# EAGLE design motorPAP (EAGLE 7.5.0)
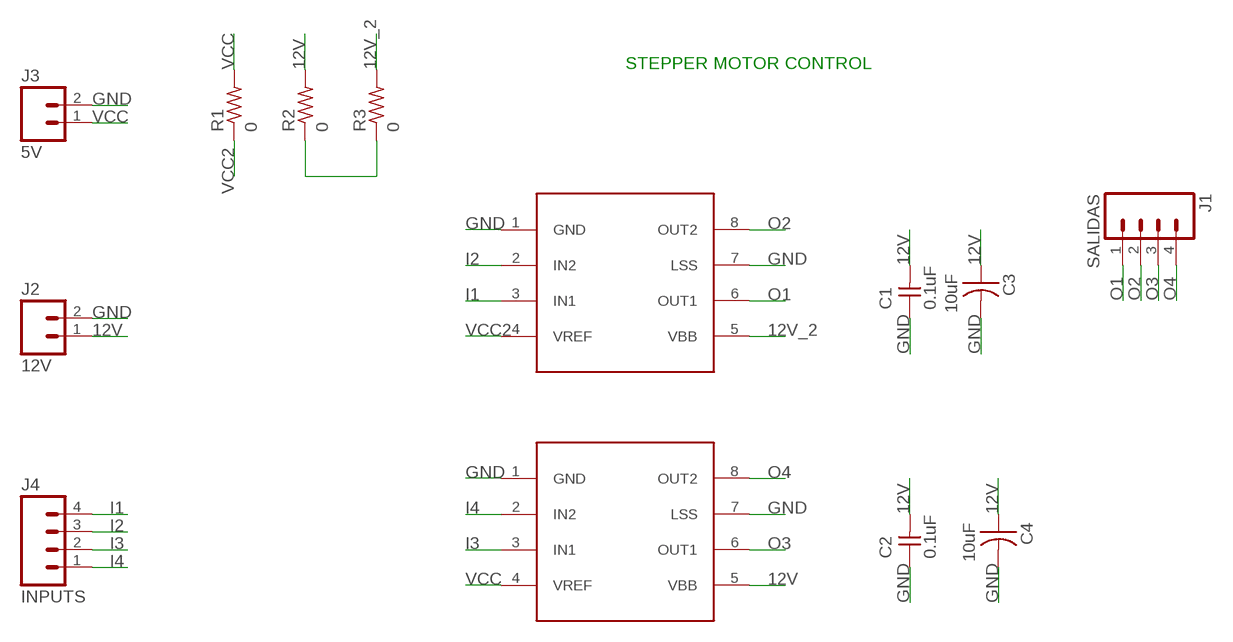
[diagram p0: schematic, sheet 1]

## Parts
C1  0.1uF  CAP-UNPOLARIZEDFAB  [C1206FAB]
C2  0.1uF  CAP-UNPOLARIZEDFAB  [C1206FAB]
C3  10uF  CAP-US1206FAB  [C1206FAB]
C4  10uF  CAP-US1206FAB  [C1206FAB]
J1  SALIDAS  M04PTH  [1X04]
J2  12V  M025MM  [SCREWTERMINAL-5MM-2]
J3  5V  M02PTH  [1X02]
J4  INPUTS  M04PTH  [1X04]
R1  0  RES-US1206FAB  [R1206FAB]
R2  0  RES-US1206FAB  [R1206FAB]
R3  0  RES-US1206FAB  [R1206FAB]
U$1  A4953-H-BRIDGE-MOTOR-DRIVER  [SOIC8]
U$2  A4953-H-BRIDGE-MOTOR-DRIVER  [SOIC8]

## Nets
12V: C1.2 C2.2 C3.1 C4.1 J2.1 R2.2 U$2.5(VBB)
12V_2: R3.2 U$1.5(VBB)
GND: C1.1 C2.1 C3.2 C4.2 J2.2 J3.2 U$1.1(GND) U$1.7(LSS) U$2.1(GND) U$2.7(LSS)
I1: J4.4 U$1.3(IN1)
I2: J4.3 U$1.2(IN2)
I3: J4.2 U$2.3(IN1)
I4: J4.1 U$2.2(IN2)
N$1: R2.1 R3.1
O1: J1.1 U$1.6(OUT1)
O2: J1.2 U$1.8(OUT2)
O3: J1.3 U$2.6(OUT1)
O4: J1.4 U$2.8(OUT2)
VCC: J3.1 R1.2 U$2.4(VREF)
VCC2: R1.1 U$1.4(VREF)

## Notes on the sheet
- STEPPER MOTOR CONTROL

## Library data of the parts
C1 C2 = fab:CAP-UNPOLARIZED
C3 C4 = fab:CAP-US
J1 J4 = SparkFun-Connectors:M04: Header 4 Standard 4-pin 0.1" header. Use with straight break away headers (SKU : PRT-00116), right angle break away headers (PRT-00553), swiss pins (PRT-00743), machine pins (PRT-00117), and female headers (PRT-00115). Molex polarized connector foot print use with SKU : PRT-08231 with associated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; PROD_ID: CONN-09696
J2 = SparkFun-Connectors:M02: Standard 2-pin 0.1" header. Use with; STOREFRONT_ID: PRT-08432
J3 = SparkFun-Connectors:M02: Standard 2-pin 0.1" header. Use with
R1-R3 = fab:RES-US: Resistor (US Symbol)
U$1 U$2 = fab:A4953-H-BRIDGE-MOTOR-DRIVER

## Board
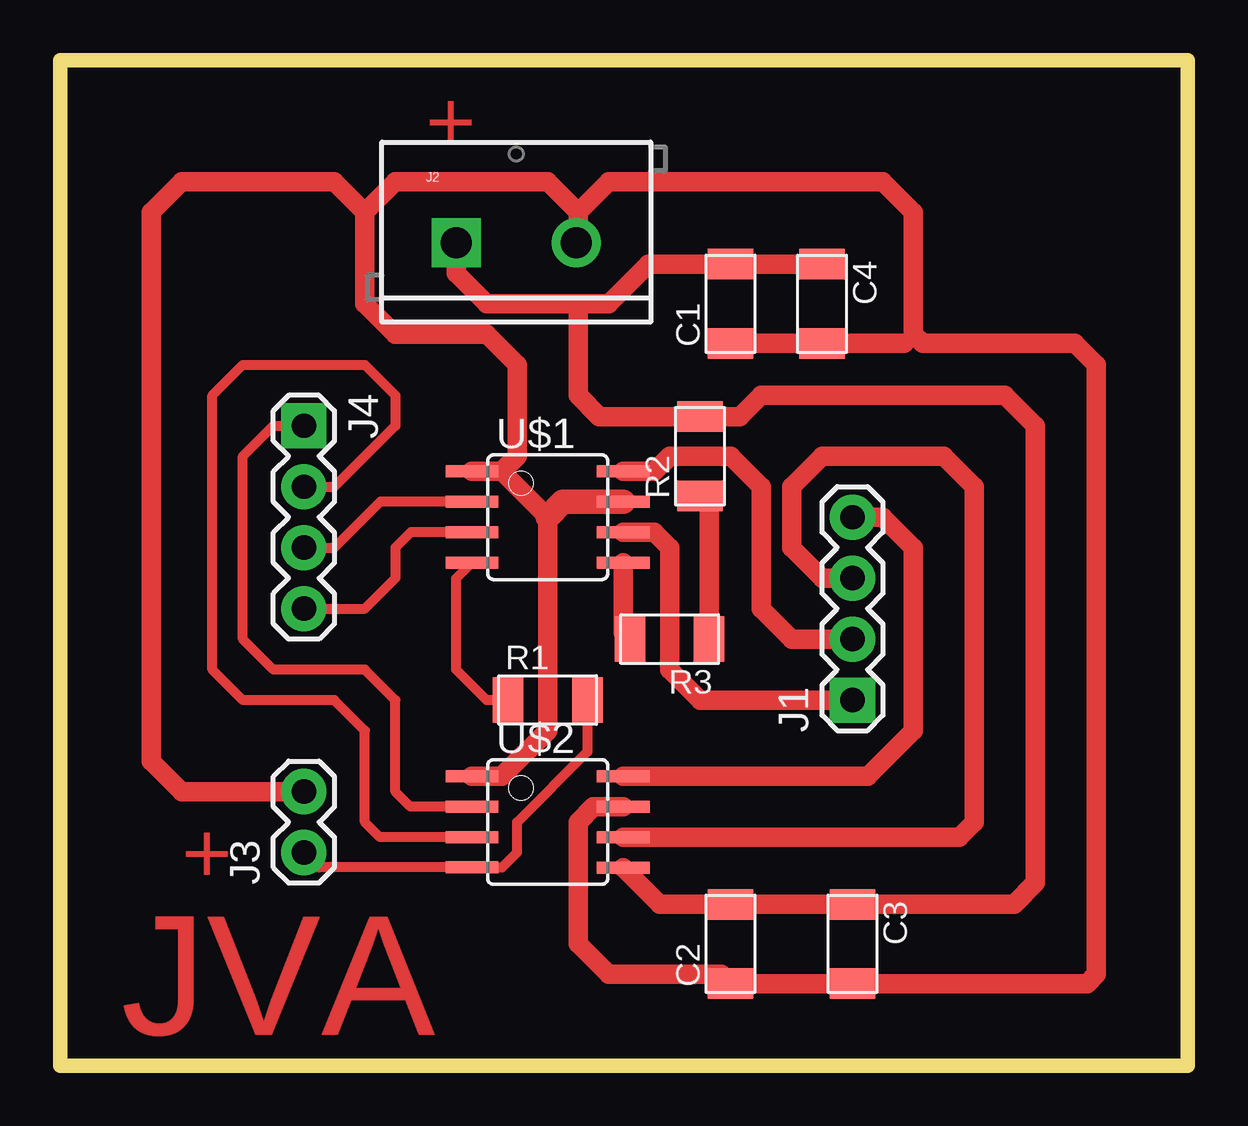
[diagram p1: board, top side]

Size 46.99 x 41.91 mm. Coordinates in mm from the lower left corner, seen from the top.
Outline: 0,41.91 46.99,41.91 46.99,0 0,0 0,41.91
Copper layers (1*16): Top 0.035mm / dielectric 1.5mm / Bottom 0.035mm
Design rules "default": minimum track width 10mil, minimum drill 24mil, track to track 8mil, track to pad 8mil, pad to pad 8mil, via to via 8mil, smd to smd 8mil, copper to edge 40mil, drill to drill 8mil, minimum pad ring 10mil, minimum via ring 8mil, stop-mask expansion 4mil, vias tented up to drill 0mil, thermal gap 10mil

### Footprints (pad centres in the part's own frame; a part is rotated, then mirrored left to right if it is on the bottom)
C1206FAB = smd 1.27 x 1.905: 1 -1.651,0; 2 1.651,0
1X04 = drill 1.016 pad 1.88 square: 1 0,0 | drill 1.016 pad 1.88: 2 2.54,0; 3 5.08,0; 4 7.62,0
SCREWTERMINAL-5MM-2 = drill 1.3 pad 2.032 square: 1 0,0 | drill 1.3 pad 2.032: 2 5,0
1X02 = drill 1.016 pad 1.88: 1 0,0; 2 2.54,0
R1206FAB = smd 1.27 x 1.905: 1 -1.651,0; 2 1.651,0
SOIC8 = smd 0.5 x 2.2: 1 -1.905,-3.154; 2 -0.645,-3.154; 3 0.625,-3.154; 4 1.895,-3.154; 5 1.905,3.154; 6 0.635,3.154; 7 -0.635,3.154; 8 -1.905,3.154

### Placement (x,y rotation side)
C1  27.94,31.75 90 top
C2  27.94,5.08 90 top
C3  33.02,5.08 270 top
C4  31.75,31.75 270 top
J1  33.02,15.24 90 top
J2  16.51,34.29 0 top
J3  10.16,8.89 90 top
J4  10.16,26.67 270 top
R1  20.32,15.24 0 top
R2  26.67,25.4 90 top
R3  25.4,17.78 180 top
U$1  20.32,22.86 270 top
U$2  20.32,10.16 270 top

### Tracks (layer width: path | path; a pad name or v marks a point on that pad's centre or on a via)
12V
  Top 0.813: U$2.5 25,6.73 C2.2 C3.1 39.75,6.73 40.64,7.62 40.64,26.67 39.37,27.94 29.21,27.94 28.32,27.05 R2.2 22.48,27.05 21.59,27.94 21.59,31.75 | C4.1 C1.2 24.51,33.4 22.86,31.75 21.59,31.75 | 21.59,31.75 17.78,31.75 16.51,33.02 J2.1
12V_2
  Top 0.813: U$1.5 23.47,18.05 R3.2
GND
  Top 0.406: 35.18,30.1 35.56,30.48
  Top 0.813: 21.59,35.56 22.86,36.83 34.29,36.83 35.56,35.56 35.56,30.48 35.94,30.1 42.29,30.1 43.18,29.21 43.18,3.81 42.8,3.43 C3.2 C2.1 27.56,3.81 22.86,3.81 21.59,5.08 21.59,10.16 22.22,10.79 U$2.7 | 35.18,30.1 C4.2 C1.1 | U$1.1 18.41,24.76 | 18.41,24.76 19.05,25.4 19.05,29.21 17.78,30.48 13.97,30.48 12.7,31.75 12.7,35.56 | 12.7,35.56 13.97,36.83 20.32,36.83 21.59,35.56 | 21.59,35.56 21.59,34.29 J2.2 | 12.7,35.56 11.43,36.83 5.08,36.83 3.81,35.56 3.81,12.7 5.08,11.43 J3.2 | 18.41,24.76 20.32,22.86 20.32,13.97 18.41,12.07 U$2.1
  Top 1.016: U$1.7 20.95,23.5 20.32,22.86
I1
  Top 0.406: U$1.3 14.61,22.24 13.97,21.59 13.97,20.32 12.7,19.05 J4.4
I2
  Top 0.406: U$1.2 13.34,23.5 11.43,21.59 J4.3
I3
  Top 0.406: U$2.3 13.32,9.54 12.7,10.16 12.7,13.97 11.43,15.24 7.62,15.24 6.35,16.51 6.35,27.94 7.62,29.21 12.7,29.21 13.97,27.94 13.97,26.67 11.43,24.13 J4.2
I4
  Top 0.406: U$2.2 14.59,10.8 13.97,11.43 13.97,15.24 12.7,16.51 8.89,16.51 7.62,17.78 7.62,25.4 8.89,26.67 J4.1
N$1
  Top 0.813: R3.1 27.05,23.37 R2.1
O1
  Top 0.813: U$1.6 24.76,22.22 25.4,21.59 25.4,16.51 26.67,15.24 J1.1
O2
  Top 0.813: J1.2 30.48,17.78 29.21,19.05 29.21,24.13 27.94,25.4 25.4,25.4 24.76,24.76 U$1.8
O3
  Top 0.813: U$2.6 37.47,9.53 38.1,10.16 38.1,24.13 36.83,25.4 31.75,25.4 30.48,24.13 30.48,21.59 31.75,20.32 J1.3
O4
  Top 0.813: J1.4 34.29,22.86 35.56,21.59 35.56,13.97 33.66,12.07 U$2.8
VCC
  Top 0.406: J3.1 10.79,8.26 U$2.4 18.43,8.26 19.05,8.89 19.05,10.16 21.97,13.08 R1.2
VCC2
  Top 0.406: R1.1 17.78,15.24 16.51,16.51 16.51,20.31 U$1.4

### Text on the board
Top: + | + | JVA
